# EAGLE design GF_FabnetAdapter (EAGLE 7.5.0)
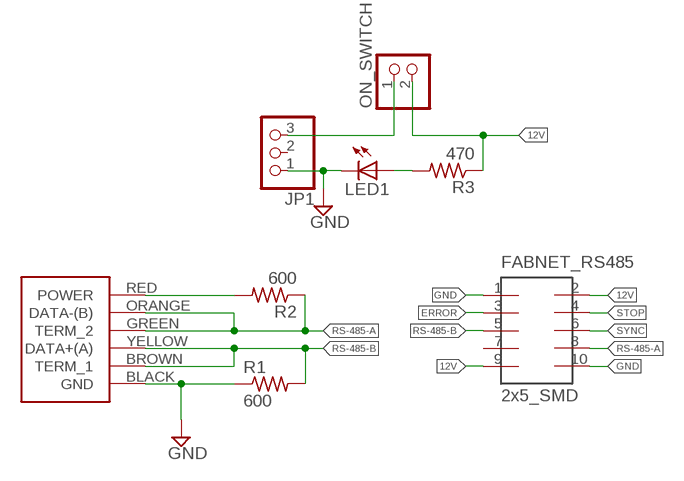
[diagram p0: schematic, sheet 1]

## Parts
FABNET_RS485  2x5_SMD  2X5HEADER  [2X5_SMD]
JP1  PINHD-1X3  [1X03]
LED1  LEDCHIPLED_1206  [CHIPLED_1206]
ON_SWITCH  PINHD-1X2  [1X02]
R1  600  R-US_R1206  [R1206]
R2  600  R-US_R1206  [R1206]
R3  470  R-US_R1206  [R1206]
U$1  USB-RS485-WE  [USB-RS485-WE]

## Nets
12V: FABNET_RS485.2 FABNET_RS485.9 ON_SWITCH.2 R3.1
ERROR: FABNET_RS485.3
GND: FABNET_RS485.1 FABNET_RS485.10 JP1.1 LED1.C R1.1 U$1.BLACK(GND)
N$1: LED1.A R3.2
N$2: R2.2 U$1.RED(POWER)
N$8: JP1.3 ON_SWITCH.1
RS-485-A: FABNET_RS485.8 R2.1 U$1.GREEN(TERM_2) U$1.ORANGE(DATA-(B))
RS-485-B: FABNET_RS485.5 R1.2 U$1.BROWN(TERM_1) U$1.YELLOW(DATA+(A))
STOP: FABNET_RS485.4
SYNC: FABNET_RS485.6
Unconnected: FABNET_RS485.7 JP1.2

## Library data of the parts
FABNET_RS485 = mellis:2X5HEADER
JP1 = pinhead:PINHD-1X3: PIN HEADER
LED1 = led:LED: LED
ON_SWITCH = pinhead:PINHD-1X2: PIN HEADER
R1-R3 = rcl:R-US_: RESISTOR, American symbol
U$1 = mellis:USB-RS485-WE

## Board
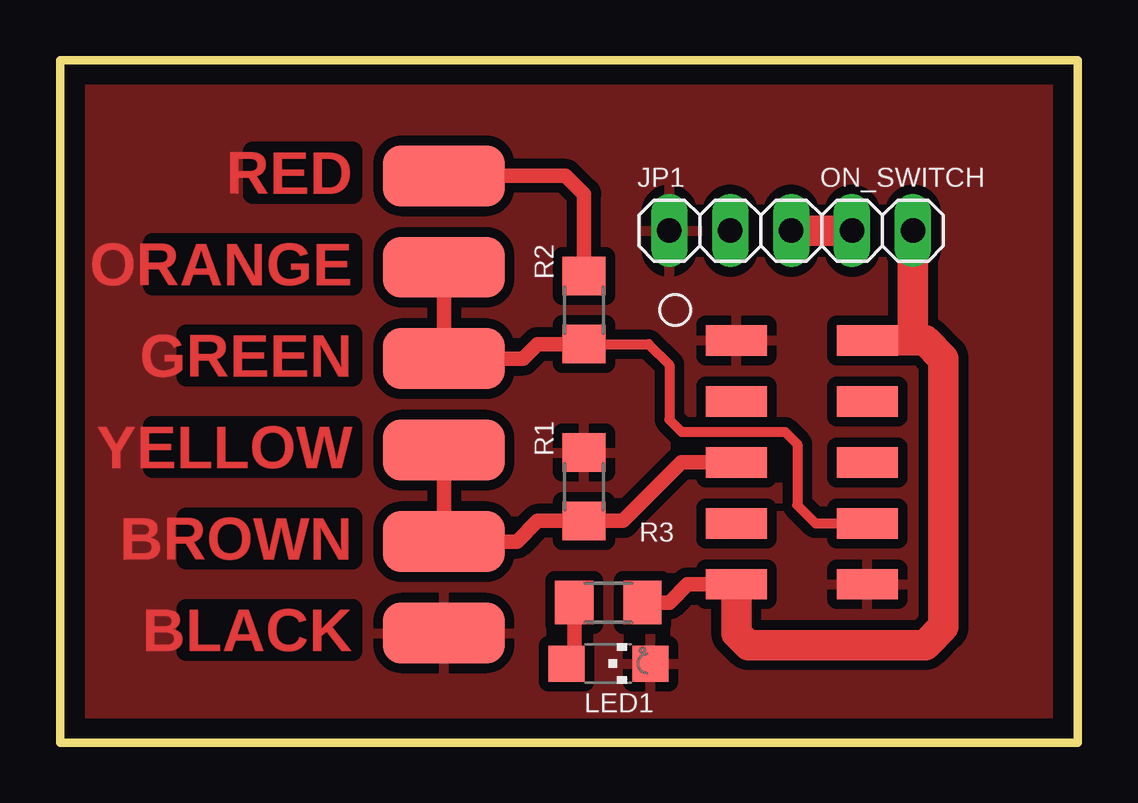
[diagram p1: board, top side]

Size 42.42 x 28.45 mm. Coordinates in mm from the lower left corner, seen from the top.
Outline: 0,0 42.42,0 42.42,28.45 0,28.45 0,0
Copper layers (1*16): Top 0.035mm / dielectric 1.5mm / Bottom 0.035mm
Design rules "default *": minimum track width 10mil, minimum drill 24mil, track to track 16mil, track to pad 16mil, pad to pad 16mil, via to via 16mil, smd to smd 16mil, copper to edge 40mil, drill to drill 8mil, minimum pad ring 10mil, minimum via ring 8mil, stop-mask expansion 4mil, vias tented up to drill 0mil, thermal gap 16mil
Milling: 4 lines

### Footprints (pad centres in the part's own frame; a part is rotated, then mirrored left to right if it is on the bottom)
2X5_SMD = smd 2.54 x 1.27: 1 -2.54,5.08; 2 2.92,5.08; 3 -2.54,2.54; 4 2.92,2.54; 5 -2.54,0; 6 2.92,0; 7 -2.54,-2.54; 8 2.92,-2.54; 9 -2.54,-5.08; 10 2.92,-5.08
1X03 = drill 1.016 long: 1 -2.54,0; 2 0,0; 3 2.54,0
CHIPLED_1206 = smd 1.5 x 1.5: A 0,-1.75; C 0,1.75
1X02 = drill 1.016 long: 1 -1.27,0; 2 1.27,0
R1206 = smd 1.6 x 1.803: 1 -1.422,0; 2 1.422,0
USB-RS485-WE = smd 5.08 x 2.54: BLACK 0,-10.16; BROWN 0,-6.35; GREEN 0,1.27; ORANGE 0,5.08; RED 0,8.89; YELLOW 0,-2.54

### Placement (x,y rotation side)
FABNET_RS485  30.73,11.68 0 top
JP1  27.94,21.34 0 top
LED1  22.86,3.3 270 top
ON_SWITCH  34.29,21.34 0 top
R1  21.84,10.67 270 top
R2  21.84,18.03 90 top
R3  22.86,5.84 180 top
U$1  16,14.73 0 top

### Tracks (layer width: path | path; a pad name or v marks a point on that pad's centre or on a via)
12V
  Top 0.61: R3.1 25.4,5.84 26.16,6.6 FABNET_RS485.9
  Top 1.27: FABNET_RS485.2 35.81,16.76 | 35.81,16.76 36.07,16.76 36.83,16 36.83,4.83 36.07,4.06 28.7,4.06 28.19,4.57 FABNET_RS485.9 | ON_SWITCH.2 35.56,17.02 35.81,16.76
GND
  pour Top (isolate 0.406): 0,0 42.42,0 42.42,28.45 0,28.45
N$1
  Top 0.61: R3.2 21.44,3.63 LED1.A
N$2
  Top 0.61: R2.2 21.84,22.86 21.08,23.62 U$1.RED
N$8
  Top 1.27: JP1.3 ON_SWITCH.1
RS-485-A
  Top 0.406: R2.1 24.54,16.61 25.4,15.75 25.4,13.46 25.91,12.95 30.23,12.95 30.73,12.45 30.73,9.91 31.5,9.14 FABNET_RS485.8
  Top 0.61: U$1.ORANGE U$1.GREEN 19.3,16 19.91,16.61 R2.1
RS-485-B
  Top 0.61: U$1.YELLOW U$1.BROWN 19.05,8.38 19.91,9.25 R1.2 23.47,9.25 25.91,11.68 FABNET_RS485.5

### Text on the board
Top: RED | ORANGE | GREEN | YELLOW | BROWN | BLACK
